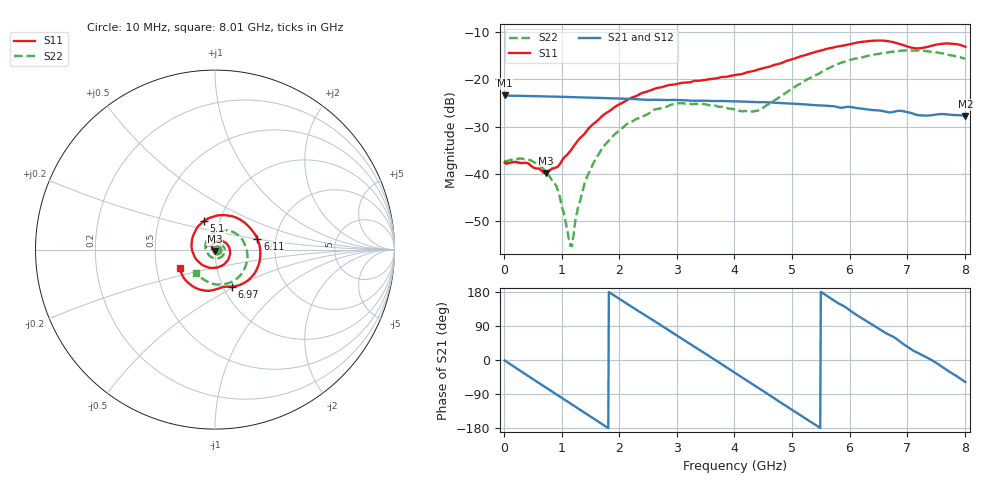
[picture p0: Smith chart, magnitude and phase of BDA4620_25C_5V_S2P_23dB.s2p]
!Agilent Technologies,E5071B,MY42404982,A.09.10
!Date: Wed May 06 09:03:21 2026
!Data & Calibration Information:
!Freq	S11:SOLT2(ON)	S21:SOLT2(ON)	S12:SOLT2(ON)	S22:SOLT2(ON)
# Hz S RI R 50
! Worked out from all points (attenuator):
!   801 points, 10 MHz to 8.01 GHz, reference 50 ohm
!   highest |S21| = -23.40 dB at 10 MHz (marker M1); lowest = -27.8 dB at 8.01 GHz (marker M2)
!   lowest |S11| = -39.8 dB at 720 MHz (marker M3), VSWR 1.02, Z = 49.8 - j0.993 ohm
!   |S11| at or under -10 dB: start of sweep to end of sweep
!   |S22| runs from -55.3 to -13.9 dB; largest |S21 - S12| = 0.00035
!   S11 on the Smith chart (normalised r, x): 10 MHz: 1.03, -0.00; 5.1 GHz: 0.84, +0.28; 6.11 GHz: 1.60, +0.21; 6.97 GHz: 1.10, -0.48; 8.01 GHz: 0.66, -0.15
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1e7  0.0132 -0.000843  0.0676 -0.00142  0.0677 -0.00143  0.0136 -0.000442
4.4e8  0.00825 -0.0096  0.0476 -0.0465  0.0477 -0.0466  0.0132 -0.00493
7.2e8  -0.00214 -0.00998  0.0202 -0.0628  0.0202 -0.0629  0.00832 -0.00695
9.3e8  -0.0106 -0.00531  -0.00343 -0.0654  -0.00352 -0.0656  0.00343 -0.00591
1.16e9  -0.0168 0.00595  -0.0282 -0.0584  -0.0284 -0.0585  -0.00153 -0.000801
1.19e9  -0.0172 0.0077  -0.0312 -0.0568  -0.0313 -0.0569  -0.00197 8.96e-05
1.26e9  -0.0179 0.0122  -0.0377 -0.0525  -0.0378 -0.0526  -0.00304 0.00221
1.35e9  -0.0174 0.0178  -0.0452 -0.0459  -0.0452 -0.0459  -0.00346 0.00495
1.56e9  -0.0114 0.0322  -0.058 -0.0268  -0.058 -0.0268  -0.003 0.013
1.83e9  0.00633 0.0456  -0.0631 0.00185  -0.0632 0.00186  0.00294 0.0227
2.15e9  0.0377 0.048  -0.0522 0.034  -0.0522 0.0341  0.0175 0.0294
2.68e9  0.0813 0.00604  -0.00623 0.0604  -0.00613 0.0605  0.0448 0.0191
3.08e9  0.076 -0.0512  0.0329 0.0505  0.0331 0.0505  0.0554 -0.00785
4.01e9  -0.0731 -0.0838  0.0486 -0.0327  0.0487 -0.0328  -0.0111 -0.0468
4.43e9  -0.1279 -0.00311  0.0148 -0.0554  0.0148 -0.0556  -0.0457 -0.0116
5.1e9  -0.06 0.1603  -0.0428 -0.0344  -0.043 -0.0344  -0.0186 0.0852
5.35e9  0.0143 0.19  -0.052 -0.0132  -0.052 -0.0132  0.0233 0.1029
6.11e9  0.2359 0.0611  -0.025 0.0432  -0.0251 0.0434  0.1613 0.0396
6.68e9  0.1907 -0.1663  0.0175 0.0413  0.0176 0.0413  0.1706 -0.0907
6.97e9  0.0932 -0.2058  0.0357 0.0281  0.0358 0.0282  0.131 -0.1537
7.6e9  -0.0794 -0.224  0.041 -0.0129  0.0411 -0.0129  -0.0231 -0.1876
8.01e9  -0.1951 -0.1046  0.0215 -0.0347  0.0217 -0.0347  -0.104 -0.1281
